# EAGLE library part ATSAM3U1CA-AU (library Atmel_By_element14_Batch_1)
AT91ARM Cortex M3-based Microcontrollers
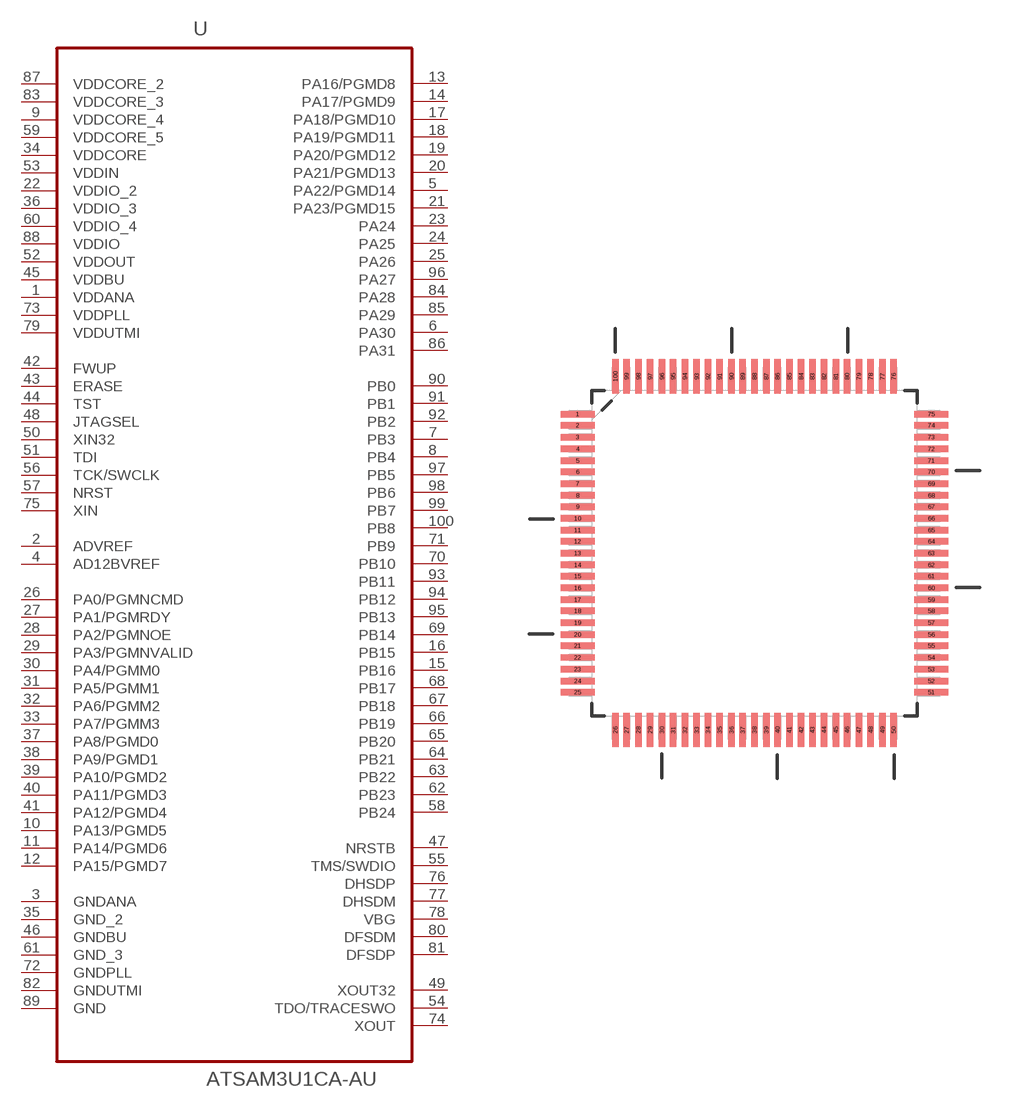
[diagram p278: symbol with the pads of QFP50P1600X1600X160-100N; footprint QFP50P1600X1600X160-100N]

Designator prefix U

## ATSAM3U1CA-AU (DESCRIPTION: AT91ARM Cortex M3-based Microcontrollers; MPN: ATSAM3U1CA-AU; OC_FARNELL: 1841659; OC_NEWARK: 12T1316; PACKAGE: LQFP-100; SUPPLIER: Atmel Corporation)  [QFP50P1600X1600X160-100N]
1  VDDANA  pwr
2  ADVREF  pas
3  GNDANA  pas
4  AD12BVREF  pas
5  PA22/PGMD14
6  PA30
7  PB3
8  PB4
9  VDDCORE_4  pwr
10  PA13/PGMD5
11  PA14/PGMD6
12  PA15/PGMD7
13  PA16/PGMD8
14  PA17/PGMD9
15  PB16
16  PB15
17  PA18/PGMD10
18  PA19/PGMD11
19  PA20/PGMD12
20  PA21/PGMD13
21  PA23/PGMD15
22  VDDIO_2  pwr
23  PA24
24  PA25
25  PA26
26  PA0/PGMNCMD
27  PA1/PGMRDY
28  PA2/PGMNOE
29  PA3/PGMNVALID
30  PA4/PGMM0
31  PA5/PGMM1
32  PA6/PGMM2
33  PA7/PGMM3
34  VDDCORE  pwr
35  GND_2  pas
36  VDDIO_3  pwr
37  PA8/PGMD0
38  PA9/PGMD1
39  PA10/PGMD2
40  PA11/PGMD3
41  PA12/PGMD4
42  FWUP  in
43  ERASE  in
44  TST  in
45  VDDBU  pwr
46  GNDBU  pas
47  NRSTB
48  JTAGSEL  in
49  XOUT32  out
50  XIN32  in
51  TDI  in
52  VDDOUT  pwr
53  VDDIN  pwr
54  TDO/TRACESWO  out
55  TMS/SWDIO
56  TCK/SWCLK  in
57  NRST  in
58  PB24
59  VDDCORE_5  pwr
60  VDDIO_4  pwr
61  GND_3  pas
62  PB23
63  PB22
64  PB21
65  PB20
66  PB19
67  PB18
68  PB17
69  PB14
70  PB10
71  PB9
72  GNDPLL  pas
73  VDDPLL  pwr
74  XOUT  out
75  XIN  in
76  DHSDP
77  DHSDM
78  VBG
79  VDDUTMI  pwr
80  DFSDM
81  DFSDP
82  GNDUTMI  pas
83  VDDCORE_3  pwr
84  PA28
85  PA29
86  PA31
87  VDDCORE_2  pwr
88  VDDIO  pwr
89  GND  pas
90  PB0
91  PB1
92  PB2
93  PB11
94  PB12
95  PB13
96  PA27
97  PB5
98  PB6
99  PB7
100  PB8

## Footprint QFP50P1600X1600X160-100N (pad centres in mm)
smd 1.473 x 0.279: 1 -7.62,5.994; 2 -7.62,5.512; 3 -7.62,5.004; 4 -7.62,4.496; 5 -7.62,3.988; 6 -7.62,3.505; 7 -7.62,2.997; 8 -7.62,2.489; 9 -7.62,2.007; 10 -7.62,1.499; 11 -7.62,0.991; 12 -7.62,0.508; 13 -7.62,0; 14 -7.62,-0.508; 15 -7.62,-0.991; 16 -7.62,-1.499; 17 -7.62,-2.007; 18 -7.62,-2.489; 19 -7.62,-2.997; 20 -7.62,-3.505; 21 -7.62,-3.988; 22 -7.62,-4.496; 23 -7.62,-5.004; 24 -7.62,-5.512; 25 -7.62,-5.994; 51 7.62,-5.994; 52 7.62,-5.512; 53 7.62,-5.004; 54 7.62,-4.496; 55 7.62,-3.988; 56 7.62,-3.505; 57 7.62,-2.997; 58 7.62,-2.489; 59 7.62,-2.007; 60 7.62,-1.499; 61 7.62,-0.991; 62 7.62,-0.508; 63 7.62,0; 64 7.62,0.508; 65 7.62,0.991; 66 7.62,1.499; 67 7.62,2.007; 68 7.62,2.489; 69 7.62,2.997; 70 7.62,3.505; 71 7.62,3.988; 72 7.62,4.496; 73 7.62,5.004; 74 7.62,5.512; 75 7.62,5.994
smd 0.279 x 1.473: 26 -5.994,-7.62; 27 -5.512,-7.62; 28 -5.004,-7.62; 29 -4.496,-7.62; 30 -3.988,-7.62; 31 -3.505,-7.62; 32 -2.997,-7.62; 33 -2.489,-7.62; 34 -2.007,-7.62; 35 -1.499,-7.62; 36 -0.991,-7.62; 37 -0.508,-7.62; 38 0,-7.62; 39 0.508,-7.62; 40 0.991,-7.62; 41 1.499,-7.62; 42 2.007,-7.62; 43 2.489,-7.62; 44 2.997,-7.62; 45 3.505,-7.62; 46 3.988,-7.62; 47 4.496,-7.62; 48 5.004,-7.62; 49 5.512,-7.62; 50 5.994,-7.62; 76 5.994,7.62; 77 5.512,7.62; 78 5.004,7.62; 79 4.496,7.62; 80 3.988,7.62; 81 3.505,7.62; 82 2.997,7.62; 83 2.489,7.62; 84 2.007,7.62; 85 1.499,7.62; 86 0.991,7.62; 87 0.508,7.62; 88 0,7.62; 89 -0.508,7.62; 90 -0.991,7.62; 91 -1.499,7.62; 92 -2.007,7.62; 93 -2.489,7.62; 94 -2.997,7.62; 95 -3.505,7.62; 96 -3.988,7.62; 97 -4.496,7.62; 98 -5.004,7.62; 99 -5.512,7.62; 100 -5.994,7.62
